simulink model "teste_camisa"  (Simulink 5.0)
settings: Solver=ode45  StartTime=0.0  StopTime=1000  MaxStep=0.002  RelTol=1e-3
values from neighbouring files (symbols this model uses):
  cPa = 1.0    (= 1)    [dados_19_2.m]
  hv_tab = [2706.3 2708.5 2710.6 2712.6 2714.5 2716.4 2718.2 2719.9 2721.5 2723.1 2724.7            2726.1 2727.6 2729.0 2730.0 2731.6]*0.2388459    [dados_19_2.m]
  Pv_alim = 2.461    [dados_19_2.m]
  Pv_tab = [   2.0    2.1    2.2    2.3    2.4    2.5    2.6    2.7    2.8    2.9    3.0               3.1    3.2    3.3    3.4    3.5]*1.019716    [dados_19_2.m]
  rhov_tab = [1/0.8854 1/0.8459 1/0.8098 1/0.7768 1/0.7465 1/0.7184 1/0.6925 1/0.6684 1/0.6460            1/0.6251 1/0.6056 1/0.5872 1/0.5700 1/0.5538 1/0.5385 1/0.5240]    [dados_19_2.m]
  Tv_tab = [120.23 121.78 123.27 124.71 126.09 127.43 128.73 129.98 131.20 132.39 133.54            134.66 135.75 136.82 137.86 138.87]    [dados_19_2.m]
  Vcam = 0.5332    [dados_19_2.m]

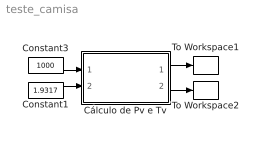
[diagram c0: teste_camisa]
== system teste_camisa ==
  Constant1 : Constant  Value=1.9317
  Constant3 : Constant  Value=1000
  Cálculo de Pv e Tv : Subsystem
  To Workspace1 : ToWorkspace  VariableName=Tv  SampleTime=-1  SaveFormat=Array
  To Workspace2 : ToWorkspace  VariableName=Pv  SampleTime=-1  SaveFormat=Array
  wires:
  Cálculo de Pv e Tv/1(Tv) -> To Workspace1/1
  Cálculo de Pv e Tv/2(Pv) -> To Workspace2/1
  Constant3/1 -> Cálculo de Pv e Tv/1(qvp)
  Constant1/1 -> Cálculo de Pv e Tv/2(Wv)

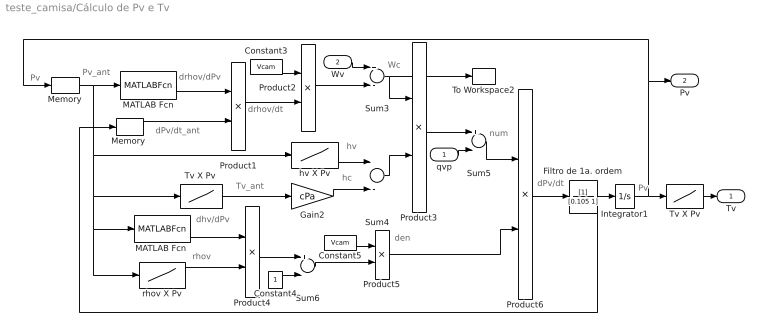
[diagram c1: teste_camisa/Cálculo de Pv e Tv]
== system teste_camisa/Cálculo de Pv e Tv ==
  note: Wc
  note: Pv_ant
  note: drhov/dPv
  note: dPv/dt_ant
  note: drhov/dt
  note: hv
  note: Tv_ant
  note: hc
  note: dhv/dPv
  note: Pv
  note: rhov
  note: den
  note: num
  note: dPv/dt
  note: Pv
  qvp : Inport
  Wv : Inport  Port=2
  Constant3 : Constant  Value=Vcam
  Constant4 : Constant
  Constant5 : Constant  Value=Vcam
  Filtro de 1a. ordem : TransferFcn  Denominator=[0.105 1]
  Gain2 : Gain  Gain=cPa
  Integrator1 : Integrator  InitialCondition=Pv_alim
  MATLAB Fcn : MATLABFcn  MATLABFcn=drhov_dPv
  "MATLAB Fcn " : MATLABFcn  MATLABFcn=dhv_dPv
  Memory : Memory  X0=Pv_alim
  "Memory " : Memory
  Product{1..5} (5 alike) : Product
  Product6 : Product  Inputs=*/
  Sum{3..6} (4 alike) : Sum  Inputs=+-
  To Workspace2 : ToWorkspace  VariableName=Wc  SampleTime=-1  SaveFormat=Array
  Tv X Pv : Lookup  InputValues=Pv_tab  OutputValues=Tv_tab
  "Tv X Pv " : Lookup  InputValues=Pv_tab  OutputValues=Tv_tab
  hv X Pv : Lookup  InputValues=Pv_tab  OutputValues=hv_tab
  rhov X Pv : Lookup  InputValues=Pv_tab  OutputValues=rhov_tab
  Tv : Outport
  Pv : Outport  Port=2
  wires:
  Wv/1 -> Sum3/1
  Memory/1 -> MATLAB Fcn/1, hv X Pv/1, rhov X Pv/1, "MATLAB Fcn "/1, "Tv X Pv "/1
  MATLAB Fcn/1 -> Product1/1
  "Memory "/1 -> Product1/2
  Product1/1 -> Product2/2
  Sum3/1 -> To Workspace2/1, Product3/1
  Constant3/1 -> Product2/1
  Product2/1 -> Sum3/2
  hv X Pv/1 -> Sum4/1
  "Tv X Pv "/1 -> Gain2/1
  Gain2/1 -> Sum4/2
  Sum4/1 -> Product3/2
  Product3/1 -> Sum5/1
  qvp/1 -> Sum5/2
  "MATLAB Fcn "/1 -> Product4/1
  rhov X Pv/1 -> Product4/2
  Product4/1 -> Sum6/1
  Constant4/1 -> Sum6/2
  Sum6/1 -> Product5/2
  Constant5/1 -> Product5/1
  Product5/1 -> Product6/2
  Sum5/1 -> Product6/1
  Product6/1 -> Filtro de 1a. ordem/1
  Integrator1/1 -> Memory/1, Pv/1, Tv X Pv/1
  Tv X Pv/1 -> Tv/1
  Filtro de 1a. ordem/1 -> Integrator1/1, "Memory "/1
